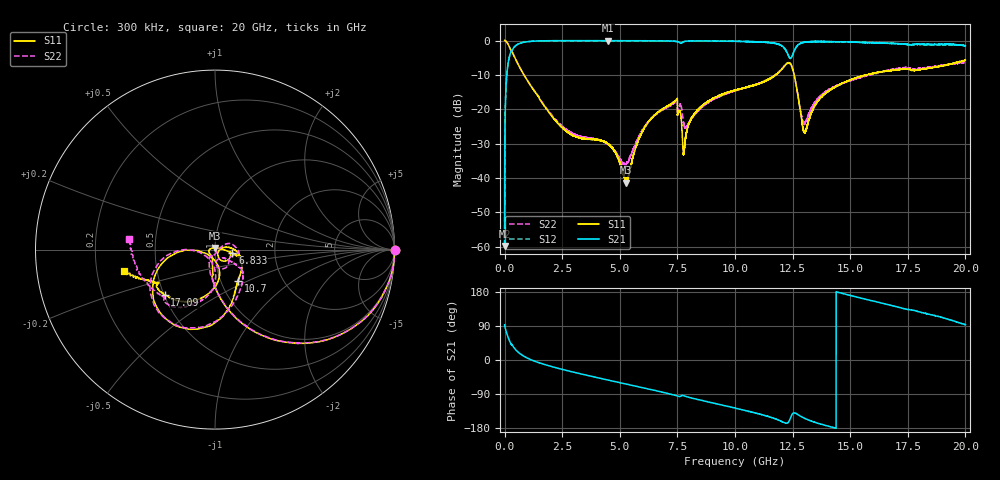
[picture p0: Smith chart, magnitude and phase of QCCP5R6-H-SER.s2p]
!QCCP5R6
!Johanson Technology Inc.
!www.johansontechnology.com
!Test Board Conditions:
!Substrate Type  RO4350B
!Substrate Thickness  20 mil
!Substrate Dk  3.66
!TL Type: GCPW
!TL Trace Width  36 mil
!TL Gap  12 mil
!Electrode orientation  Horizontal
!DUT TOPOLOGY	SERIES
!Mounting Pad LxW  26x36 mil
# MHz S  dB  R 50
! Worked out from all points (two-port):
!   20001 points, 300 kHz to 20 GHz, reference 50 ohm
!   highest |S21| = -0.03 dB at 4.491 GHz (marker M1); lowest = -59.8 dB at 300 kHz (marker M2)
!   |S21| within 3 dB of the highest: 312.5 MHz to 12.22 GHz (11.91 GHz wide, 190 % of centre); 12.57 GHz to end of sweep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
!   lowest |S11| = -41.4 dB at 5.252 GHz (marker M3), VSWR 1.02, Z = 49.9 + j0.843 ohm
!   |S11| at or under -10 dB: 839.5 MHz to 11.78 GHz (10.94 GHz wide, 173 % of centre); 12.57 GHz to 15.67 GHz (3.107 GHz wide, 22 % of centre); 15.67563 GHz to 15.68285 GHz (7.217 MHz wide, 0.046 % of centre)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
!   |S22| runs from -36.5 to 0.0 dB; largest |S21 - S12| = 0.043
!   S11 on the Smith chart (normalised r, x): 300 kHz: open; 6.833 GHz: 1.21, -0.05; 10.7 GHz: 1.21, -0.44; 17.09 GHz: 0.50, -0.30; 20 GHz: 0.32, -0.11
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0.3  0.00 -0.1  -59.82 93.1  -59.90 85.0  0.01 -0.1
114.298  -0.64 -22.9  -8.66 66.7  -8.67 66.9  -0.63 -23.0
328.295  -3.33 -49.8  -2.83 39.7  -2.82 39.8  -3.34 -49.7
1103.283  -12.86 -87.9  -0.27 1.8  -0.26 1.7  -12.80 -87.8
3334.25  -28.50 -129.6  -0.04 -37.0  -0.04 -37.0  -28.05 -121.9
4491.233  -30.20 180.0  -0.03 -52.9  -0.04 -52.9  -30.25 -98.8
5252.221  -41.36 98.7  -0.05 -63.2  -0.04 -63.2  -36.49 -33.7
6667.2  -20.83 -10.5  -0.09 -82.4  -0.11 -82.5  -20.98 22.4
6833.198  -20.07 -12.2  -0.11 -84.6  -0.11 -84.7  -20.36 19.5
7399.189  -17.62 -14.9  -0.23 -93.3  -0.23 -93.4  -18.01 -0.2
7806.183  -31.37 -0.8  -0.26 -94.9  -0.28 -94.9  -25.01 -73.1
8414.174  -20.00 3.5  -0.12 -104.5  -0.11 -104.6  -20.30 -36.9
10000.15  -14.46 -39.6  -0.21 -126.8  -0.23 -126.7  -14.69 -37.1
10698.14  -13.27 -53.6  -0.31 -137.1  -0.34 -136.7  -13.11 -44.5
11891.12  -9.36 -77.6  -1.10 -158.7  -1.09 -159.0  -9.19 -78.0
12350.11  -6.46 -122.6  -4.80 -161.0  -4.87 -161.3  -6.50 -127.2
12637.11  -12.27 -172.5  -2.10 -140.6  -2.13 -140.5  -12.49 -175.8
12995.1  -26.27 -137.8  -0.53 -153.5  -0.53 -153.4  -24.29 -135.7
13334.1  -20.70 -79.8  -0.32 -161.7  -0.32 -161.8  -19.44 -91.4
16667.05  -8.84 -131.5  -0.82 145.7  -0.74 144.9  -8.61 -119.5
17086.04  -8.49 -138.0  -0.94 139.4  -0.89 138.7  -8.12 -126.2
20000  -5.64 -166.5  -1.50 93.3  -1.34 95.2  -6.32 172.6
